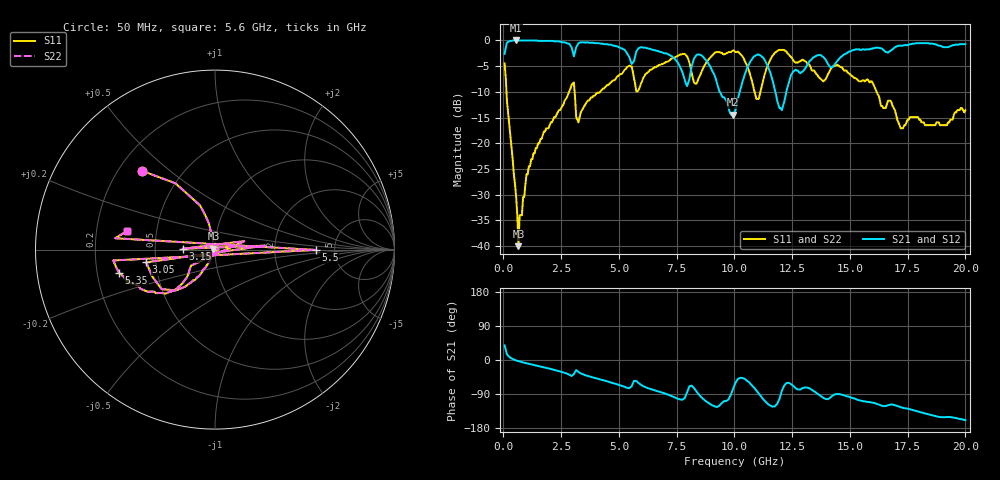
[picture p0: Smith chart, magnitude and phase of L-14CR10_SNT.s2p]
# MHZ S MA R 50
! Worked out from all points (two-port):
!   400 points, 50 MHz to 20 GHz, reference 50 ohm
!   highest |S21| = 0.00 dB at 550 MHz (marker M1); lowest = -14.4 dB at 9.95 GHz (marker M2)
!   |S21| within 3 dB of the highest: start of sweep to 3.045 GHz; 14.67 GHz to end of sweep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
!   lowest |S11| = -40.0 dB at 650 MHz (marker M3), VSWR 1.02, Z = 49.1 + j0.506 ohm
!   |S11| at or under -10 dB: 130.5 MHz to 2.841 GHz (2.71 GHz wide, 182 % of centre); 3.082 GHz to 4.181 GHz (1.1 GHz wide, 30.3 % of centre); 16.16 GHz to end of sweep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
!   |S22| runs from -40.0 to -1.8 dB; largest |S21 - S12| = 0
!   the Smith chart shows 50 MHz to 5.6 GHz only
!   S11 on the Smith chart (normalised r, x): 50 MHz: 0.29, +0.40; 3.05 GHz: 0.44, -0.07; 3.15 GHz: 0.69, +0.01; 5.35 GHz: 0.29, -0.11; 5.5 GHz: 3.55, -0.02; 5.6 GHz: 0.34, +0.09
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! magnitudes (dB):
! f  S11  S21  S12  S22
! 50 MHz  -4.4  -2.6  -2.6  -4.4
! 550 MHz  -30.5  0.0  0.0  -30.5
! 650 MHz  -40.0  0.0  0.0  -40.0
! 700 MHz  -34.0  0.0  0.0  -34.0
! 1.2 GHz  -23.1  0.0  0.0  -23.1
! 3.05 GHz  -8.2  -3.1  -3.1  -8.2
! 3.15 GHz  -14.9  -1.3  -1.3  -14.9
! 3.4 GHz  -13.6  -0.4  -0.4  -13.6
! 5.35 GHz  -5.2  -2.5  -2.5  -5.2
! 5.5 GHz  -5.0  -3.9  -3.9  -5.0
! 5.6 GHz  -6.0  -4.3  -4.3  -6.0
! 6.7 GHz  -4.9  -2.0  -2.0  -4.9
! 7.95 GHz  -3.1  -8.9  -8.9  -3.1
! 8.6 GHz  -5.8  -3.0  -3.0  -5.8
! 9.95 GHz  -1.9  -14.4  -14.4  -1.9
! 10.05 GHz  -2.3  -13.6  -13.6  -2.3
! 10.95 GHz  -11.4  -2.9  -2.9  -11.4
! 12.05 GHz  -1.8  -13.6  -13.6  -1.8
! 13.35 GHz  -5.8  -3.6  -3.6  -5.8
! 16.7 GHz  -11.7  -2.2  -2.2  -11.7
! 17.2 GHz  -17.1  -1.0  -1.0  -17.1
! 20 GHz  -13.6  -0.7  -0.7  -13.6
